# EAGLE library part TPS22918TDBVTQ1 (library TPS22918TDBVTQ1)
5.5V, 2A, 52m Automotive High-Side Load Switch with Adjustable Rise Time & Quick Output Discharge Source: Datasheet
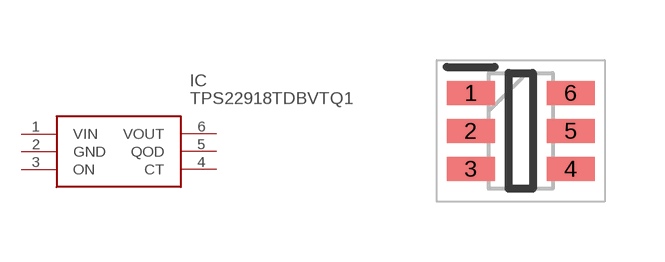
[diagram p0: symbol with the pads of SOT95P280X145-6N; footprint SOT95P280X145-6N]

Designator prefix IC

## TPS22918TDBVTQ1 (Arrow_Part_Number: TPS22918TDBVTQ1; Arrow_Price-Stock: https://www.arrow.com/en/products/tps22918tdbvtq1/texas-instruments.html?utm_currency=USD&region=nac; Description: 5.5V, 2A, 52m Automotive High-Side Load Switch with Adjustable Rise Time & Quick Output Discharge; Height: 1.45mm; Manufacturer_Name: Texas Instruments; Manufacturer_Part_Number: TPS22918TDBVTQ1; Mouser_Part_Number: 595-TPS22918TDBVTQ1; Mouser_Price-Stock: https://www.mouser.co.uk/ProductDetail/Texas-Instruments/TPS22918TDBVTQ1?qs=AvgxZrxb8y2k10t5sHUssQ%3D%3D)  [SOT95P280X145-6N]
1  VIN
2  GND
3  ON
4  CT
5  QOD
6  VOUT

## Footprint SOT95P280X145-6N (pad centres in mm)
DBV (R-PDSO-G6)
smd 1.2 x 0.6: 1 -1.25,0.95; 2 -1.25,0; 3 -1.25,-0.95; 4 1.25,-0.95; 5 1.25,0; 6 1.25,0.95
